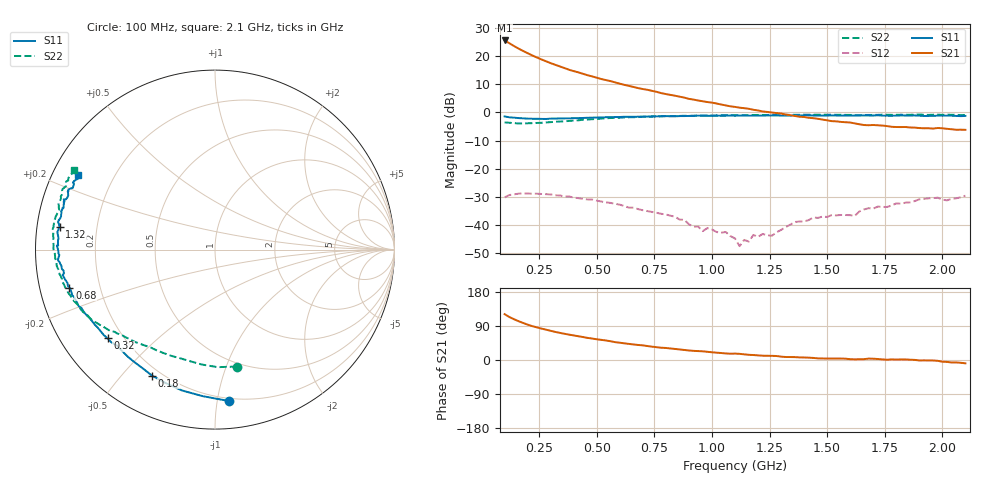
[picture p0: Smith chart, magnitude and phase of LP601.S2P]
!  POLYFET RF DEVICES
!  S PARAMETERS FOR
!  LP601
!  VDS=28, IDQ=200mA
# MHZ S MA R 50
! Freq=Mhz Mag[s11] Ang[s11] Mag[s21] Ang[s21] Mag[s12] Ang[s12] Mag[s22] Ang[s22]
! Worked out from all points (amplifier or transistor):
!   101 points, 100 MHz to 2.1 GHz, reference 50 ohm
!   highest |S21| = 25.6 dB at 100 MHz (marker M1)
!   |S21| within 3 dB of that: start of sweep to 163.1 MHz
!   unconditionally stable (mu >= 1): 896.4 MHz to end of sweep
!   at 420 MHz: K = 0.14, MSG = 22.4 dB, |S12| = -30.5 dB
!   at 1.1 GHz: K = 2.60, MAG = 16.4 dB, |S12| = -44.8 dB
!   at 2.1 GHz: K = 1.89, MAG = 6.3 dB, |S12| = -29.6 dB
!   S11 on the Smith chart (normalised r, x): 100 MHz: 0.18, -1.08; 180 MHz: 0.17, -0.61; 320 MHz: 0.14, -0.35; 680 MHz: 0.09, -0.13; 1.32 GHz: 0.07, +0.07; 2.1 GHz: 0.08, +0.25
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100  0.8479 -84.6  19.02 121.0  0.03077 33.5  0.6629 -79.4
120  0.8191 -94.9  17.03 113.6  0.03388 25.7  0.6551 -88.7
140  0.806 -103.3  15.2 107.8  0.03485 19.2  0.6444 -96.6
160  0.7925 -110.6  13.67 102.5  0.03585 15.8  0.6369 -103.0
180  0.7848 -116.6  12.39 97.8  0.03635 11.0  0.6358 -107.9
200  0.7746 -121.2  11.3 93.3  0.03602 6.1  0.6402 -112.5
240  0.7695 -129.2  9.468 86.1  0.03584 -0.0  0.6487 -120.2
280  0.7642 -135.7  8.11 80.0  0.03514 -5.4  0.6627 -126.4
320  0.776 -140.4  7.019 74.1  0.03352 -10.3  0.6818 -131.1
380  0.7845 -146.3  5.731 66.9  0.03195 -16.5  0.7041 -137.4
440  0.7959 -151.4  4.858 60.6  0.02901 -20.8  0.7401 -142.3
500  0.8098 -154.9  4.14 54.6  0.02696 -23.3  0.7664 -146.9
580  0.8266 -160.7  3.416 47.1  0.02372 -27.9  0.799 -152.8
680  0.838 -165.3  2.703 39.6  0.01903 -31.4  0.8258 -158.4
780  0.8552 -169.6  2.202 32.4  0.01574 -33.5  0.8521 -163.5
900  0.8655 -174.7  1.741 25.1  0.01025 -36.5  0.8686 -169.2
1100  0.8736 178.4  1.252 16.9  0.00574 -9.2  0.8921 -177.1
1120  0.878 178.5  1.214 16.2  0.00418 11.3  0.8919 -177.7
1320  0.8752 171.7  0.9183 7.9  0.00913 65.9  0.9023 175.8
1440  0.8808 168.8  0.7887 5.5  0.01354 77.6  0.9083 172.0
1780  0.8713 159.8  0.5548 1.6  0.02209 81.1  0.9042 162.1
2100  0.8656 151.5  0.4896 -8.7  0.03302 71.4  0.8996 150.5
